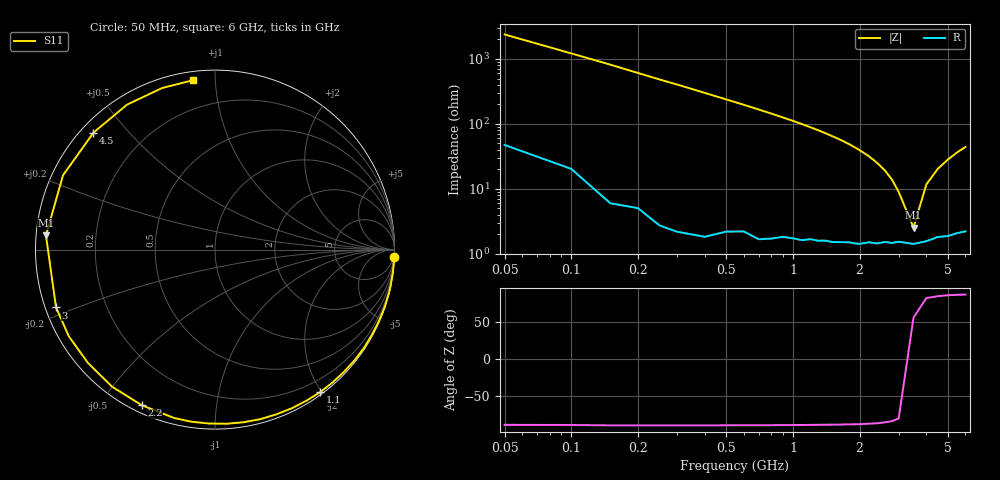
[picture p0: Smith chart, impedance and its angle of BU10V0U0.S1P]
! Infineon Technologies  Discrete & RF Semiconductors
! BB 833
! Si Tuning Diode in SOD323
! VR = 10 V
! S-Parameters:  June  1999
# GHz  S  MA  R  50
!  f  S11
! GHz  MAG  ANG
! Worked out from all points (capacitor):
!   34 points, 50 MHz to 6 GHz, reference 50 ohm
!   read as one part to ground: C = 1.31 pF near 50 MHz
!   lowest |Z| = 2.53 ohm at 3.5 GHz (marker M1)
!   series resonance near 3.404 GHz, so ESL is about 1.7 nH
!   S11 on the Smith chart (normalised r, x): 50 MHz: 1, -48; 1.1 GHz: 0.03, -1.98; 2.2 GHz: 0.03, -0.63; 3 GHz: 0.03, -0.18; 4.5 GHz: 0.04, +0.40; 6 GHz: 0.04, +0.88
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0.05  0.9992 -2.4
0.15  0.9991 -7.0
0.25  0.9989 -11.8
0.4  0.998 -18.9
0.6  0.9947 -28.5
0.7  0.9945 -33.4
0.8  0.9927 -38.3
1  0.9885 -48.4
1.1  0.987 -53.6
1.3  0.9823 -64.2
1.4  0.9795 -69.6
1.5  0.9778 -75.1
1.6  0.9751 -80.6
1.7  0.9723 -86.3
1.8  0.9695 -92.0
1.9  0.9679 -97.8
2  0.9656 -103.6
2.2  0.9582 -115.2
2.4  0.9551 -126.9
2.6  0.9485 -138.2
2.8  0.947 -149.3
3  0.9424 -160.0
3.5  0.9452 175.2
4  0.9427 153.9
4.5  0.9397 136.1
5  0.9447 121.3
5.5  0.9472 108.1
6  0.9514 97.4
